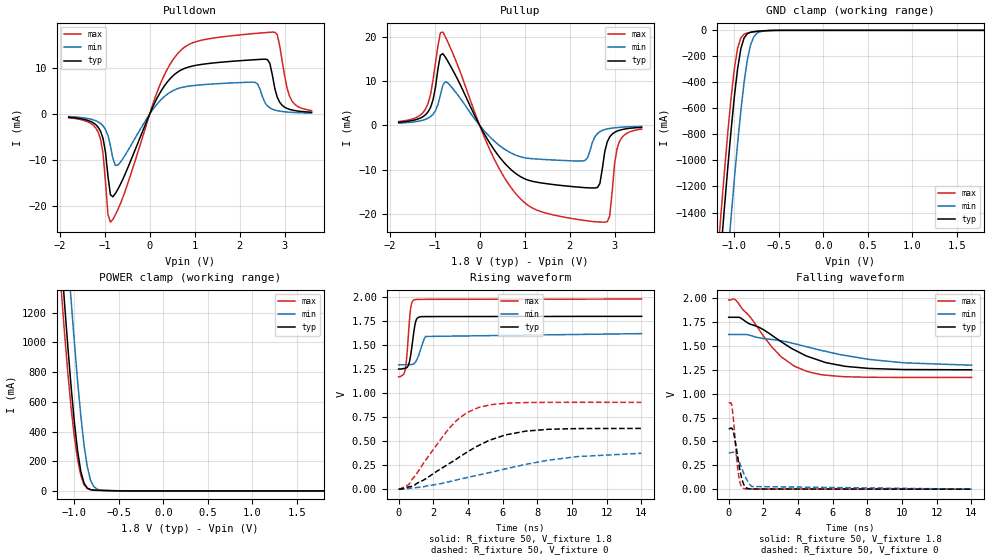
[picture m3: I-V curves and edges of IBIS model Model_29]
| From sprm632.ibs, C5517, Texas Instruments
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| Model based on original model for BC3350CTHYPD
|   Sub model PD_ON_COM_1P8
[model]   Model_29
|[Description]  [1.8V-I/O-PD-X, COM]
|   PD,COM,
|[Input Load]   PD
|[Output Drive]
|Voltage   1.8V
|Mode   I/O
Model_type   I/O
Polarity   Non-Inverting
Enable   Active-Low
Vinl =  0.63
Vinh =  1.17
Cref =  15.0000pF
Rref =  100.0000M
Vref =  0V
Vmeas =  0.9
C_comp   1.505438p   1.4840531p   1.52103p
[Model Spec]
Vinl   0.63   0.567   0.693
Vinh   1.17   1.053   1.287
[Temperature Range]   25   105   -10
[Voltage Range]   1.8   1.62   1.98
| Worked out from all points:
|   slope of the pulldown table from 0 to 0.27 V, typ, clamps not added: 51 ohm
|   slope of the pullup table from 0 to 0.27 V, typ, clamps not added: 57.1 ohm
|   GND clamp passes 1 mA (typ) near -0.58 V on its own axis
|   POWER clamp passes 1 mA (typ) near -0.52 V on its own axis
|   rising waveform, R_fixture 50, V_fixture 1.8: 20-80 % time 262ps typ, 379ps min, 208ps max; typ from 1.25 V to 1.8 V
|   rising waveform, R_fixture 50, V_fixture 0: 20-80 % time 3.48ns typ, 5.71ns min, 2.28ns max; typ from 0.001 V to 0.633 V
|   falling waveform, R_fixture 50, V_fixture 1.8: 20-80 % time 3.24ns typ, 5.02ns min, 2.28ns max; typ from 1.8 V to 1.25 V
|   falling waveform, R_fixture 50, V_fixture 0: 20-80 % time 360ps typ, 552ps min, 268ps max; typ from 0.633 V to 0 V
[POWER_clamp]
-1.8V     7.656A     8.299A     7.406A
-1.145V   1.557A     2.196A     1.339A
-1.109V   1.256A     1.883A     1.055A
-1.036V   703.1mA    1.284A     559.8mA
-963.6mV  270.2mA    740.6mA    213.7mA
-927.3mV  130.5mA    505.1mA    105.4mA
-890.9mV  51.5mA     307.4mA    41.89mA
-854.5mV  19.14mA    161.4mA    16.19mA
-818.2mV  8.562mA    72.08mA    8.402mA
-781.8mV  5.313mA    29.19mA    6.041mA
-672.7mV  2.755mA    3.311mA    3.478mA
1.8V      -3.013nA   -5.095uA   8.701uA
[Pulldown]
-1.8V     -681.9uA   -528.3uA   -799.6uA
-1.145V   -2.848mA   -1.688mA   -3.914mA
-1.036V   -5.318mA   -2.553mA   -8.567mA
-872.7mV  -17.57mA   -6.855mA   -23.59mA
-709.1mV  -16.44mA   -11.17mA   -20.89mA
272.7mV   5.341mA    3.341mA    7.405mA
872.7mV   10.3mA     6.104mA    15.2mA
2.345V    11.88mA    6.92mA     17.61mA
2.618V    11.89mA    1.797mA    17.83mA
2.782V    5.623mA    889uA      17.88mA
3.109V    1.046mA    417.7uA    3.932mA
3.6V      416.6uA    227.7uA    789.5uA
[Pullup]
-1.8V     683.6uA    489.2uA    862.2uA
-1.2V     2.423mA    1.368mA    3.724mA
-818.2mV  16.21mA    9.062mA    21.1mA
218.2mV   -3.905mA   -2.516mA   -5.325mA
872.7mV   -11.39mA   -7.011mA   -16.27mA
2.345V    -14.1mA    -7.933mA   -21.55mA
2.618V    -14.07mA   -1.864mA   -21.85mA
2.782V    -5.914mA   -955.1uA   -21.92mA
2.891V    -2.623mA   -708.3uA   -20.54mA
3V        -1.582mA   -559.9uA   -8.606mA
3.109V    -1.114mA   -461.7uA   -3.639mA
3.6V      -465.4uA   -255.6uA   -860.2uA
[GND_clamp]
-1.8V     -7.797A    -8.487A    -7.522A
-1.182V   -1.972A    -2.683A    -1.687A
-1.145V   -1.654A    -2.361A    -1.372A
-1.109V   -1.345A    -2.044A    -1.068A
-1.036V   -766.6mA   -1.434A    -516.9mA
-1V       -511.2mA   -1.144A    -295mA
-963.6mV  -296.8mA   -871.2mA   -139.2mA
-927.3mV  -142.6mA   -620.4mA   -58.96mA
-890.9mV  -58.96mA   -401.7mA   -29.75mA
-818.2mV  -14.99mA   -112.4mA   -14.94mA
-709.1mV  -5.178mA   -10.46mA   -6.012mA
1.8V      20.41uA    14.91uA    31.82uA
[Ramp]
dV/dt_f 0.33517628/3.2899718n 0.19923451/5.2308685n 0.49236419/2.3079812n
dV/dt_r 0.38012451/3.4840773n 0.22863115/5.8919992n 0.54318229/2.2860461n
R_load = 50
[Rising Waveform]
R_fixture = 50
V_fixture = 1.8
V_fixture_min = 1.62
V_fixture_max = 1.98
0s        1.251V     1.295V     1.171V
292.5ps   1.257V     1.295V     1.199V
395.6ps   1.26V      1.296V     1.263V
556.5ps   1.287V     1.296V     1.593V
675.3ps   1.377V     1.297V     1.862V
772.7ps   1.497V     1.299V     1.947V
917.6ps   1.687V     1.312V     1.973V
1.066ns   1.779V     1.356V     1.976V
1.549ns   1.797V     1.59V      1.977V
14.02ns   1.799V     1.62V      1.979V
[Rising Waveform]
R_fixture = 50
V_fixture = 0
V_fixture_min = 0
V_fixture_max = 0
0s        657.1uV    353.9uV    833.1uV
599.9ps   24.21mV    8.078mV    52.96mV
2.561ns   227mV      63.13mV    552.4mV
3.342ns   315.7mV    96.48mV    716.2mV
3.922ns   382.9mV    120.3mV    796.3mV
4.647ns   457.6mV    148.9mV    853.4mV
6.139ns   564.1mV    210.3mV    894.3mV
7.335ns   604.6mV    258.4mV    901.7mV
10.26ns   631mV      338.8mV    904.6mV
14.01ns   632.8mV    373.6mV    904.3mV
[Falling Waveform]
R_fixture = 50
V_fixture = 1.8
V_fixture_min = 1.62
V_fixture_max = 1.98
0s        1.799V     1.62V      1.979V
414.9ps   1.799V     1.62V      1.978V
1.851ns   1.685V     1.581V     1.644V
2.471ns   1.613V     1.567V     1.492V
3.036ns   1.542V     1.553V     1.385V
3.797ns   1.457V     1.523V     1.287V
4.557ns   1.389V     1.488V     1.23V
5.607ns   1.325V     1.442V     1.193V
8.115ns   1.263V     1.358V     1.171V
14.02ns   1.25V      1.298V     1.17V
[Falling Waveform]
R_fixture = 50
V_fixture = 0
V_fixture_min = 0
V_fixture_max = 0
0s        633.2mV    380.9mV    904.3mV
131ps     639.7mV    382.6mV    904.3mV
206.2ps   630.6mV    386.5mV    844.4mV
299.2ps   580.4mV    383.8mV    679.5mV
503.5ps   358.2mV    331.3mV    245.7mV
604.9ps   244.2mV    287.8mV    108.2mV
718.7ps   139.4mV    234.2mV    32.71mV
887.1ps   42.85mV    158.3mV    5.333mV
1.342ns   1.583mV    27.69mV    1.82mV
14.01ns   0V         14.65uV    0V
